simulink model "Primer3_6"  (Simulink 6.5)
settings: Solver=ode23t  SolverMode=SingleTasking  StartTime=0.0  StopTime=1  RelTol=1e-3  AbsTol=1e-2
undefined symbols (not defined in the file or in its folder): blocks, Continuous, powergui, ZData
libraries: powerlib x8, powerlib_extras x2

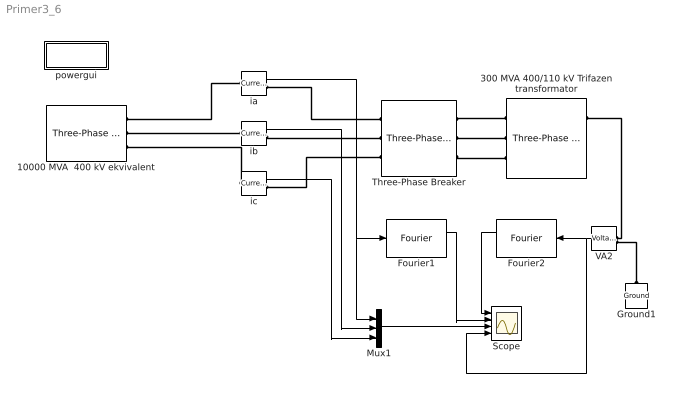
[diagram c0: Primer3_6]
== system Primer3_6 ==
  10000 MVA  400 kV ekvivalent : powerlib/Electrical Sources/Three-Phase Source  DialogController=PMDialogs.PMDefaultMaskDlg  SystemSampleTime=-1  Voltage=400e3  PhaseAngle=0  Frequency=50  InternalConnection=Yg  SpecifyImpedance=on  Resistance=5.55  Inductance=0.221  ShortCircuitLevel=10000e6  BaseVoltage=400e3  XRratio=10
  300 MVA 400/110 kV Trifazen transformator : powerlib/Elements/Three-Phase Transformer (Two Windings)  DialogController=PMDialogs.PMDefaultMaskDlg  SystemSampleTime=-1  UNITS=pu  NominalPower=[ 300e6 50 ]  Winding1Connection=Yg  Winding1=[ 400e3 0.0005 0.02 ]  Winding2Connection=Yg  Winding2=[ 115.5e3 0.0005 0.02]  SetSaturation=on  Rm=125  Lm=500  Saturation="[0 0; 0.0 1.2; 1.0  1.52]"  Hysteresis=off  DataFile='hysteresis'  SetInitialFlux=off  InitialFluxes=[-0.000666222505893204 0.000333111406701593 0.000333111099191611]  Measurements=None  TransfoNumber=0  MoreParameters=off  BreakLoop=off  DataType=off
  Fourier1 : powerlib_extras/Measurements/Fourier  DialogController=PMDialogs.PMDefaultMaskDlg  SystemSampleTime=-1  f1=50  n=3
  Fourier2 : powerlib_extras/Measurements/Fourier  Orientation=left  DialogController=PMDialogs.PMDefaultMaskDlg  SystemSampleTime=-1  f1=50  n=3
  Ground1 : powerlib/Elements/Ground  Orientation=down  DialogController=PMDialogs.PMDefaultMaskDlg  PhysicalDomain=powersysdomain  SubClassName=unknown  LeftPortType=p1  RightPortType=p1  LConnTagsString=a
  Mux1 : Mux  Inputs=3
  Scope : Scope  NumInputPorts=4
  Three-Phase Breaker : powerlib/Elements/Three-Phase Breaker  DialogController=PMDialogs.PMDefaultMaskDlg  SystemSampleTime=-1  InitialState=open  SwitchA=on  SwitchB=on  SwitchC=on  SwitchTimes=[0.05]  External=off  BreakerResistance=0.001  SnubberResistance=100e6  SnubberCapacitance=inf  Measurements=None
  VA2 : powerlib/Measurements/Voltage Measurement  Tag=PoWeRsYsTeMmEaSuReMeNt  Orientation=left  DialogController=PMDialogs.PMDefaultMaskDlg  SystemSampleTime=-1  PhasorSimulation=off  OutputType=Magnitude  PSBequivalent=0
  ia : powerlib/Measurements/Current Measurement  Tag=PoWeRsYsTeMmEaSuReMeNt  DialogController=PMDialogs.PMDefaultMaskDlg  SystemSampleTime=-1  PhasorSimulation=off  OutputType=Magnitude  PSBequivalent=0
  ib : powerlib/Measurements/Current Measurement  Tag=PoWeRsYsTeMmEaSuReMeNt  DialogController=PMDialogs.PMDefaultMaskDlg  SystemSampleTime=-1  PhasorSimulation=off  OutputType=Magnitude  PSBequivalent=0
  ic : powerlib/Measurements/Current Measurement  Tag=PoWeRsYsTeMmEaSuReMeNt  DialogController=PMDialogs.PMDefaultMaskDlg  SystemSampleTime=-1  PhasorSimulation=off  OutputType=Magnitude  PSBequivalent=0
  powergui : Subsystem  AncestorBlock=powerlib/powergui  InitFcn=powergui( 'InitFcn_Callback' , gcb , 0 , [ ] );  mask(PSB option menu block){SimulationMode=Continuous, SampleTime=0, echomessages=off, RestoreLinks=warning, x0status=blocks, Frange=[0:2:500], Ylog=off, Xlog=on, ShowGrid=off, save=off, variable=ZData, structure=, ZoomFFT=on, StartTime=0.0, cycles=1, DisplayStyle=1, fundamental=60, FreqAxis=off, MaxFrequency=1000, frequencyindice=50, frequencyindicesteady=1, RmsSteady=1, display=off, Ts=0, frequency=60, methode=off, HookPort=off, Interpol=off}
      mask prompts: SimulationMode "Simulation mode"; SampleTime "Sample time Ts (when simulation mode is Discrete) (s)"; echomessages "Echo  Messages"; RestoreLinks "Restore disabled links"; x0status "Initial electrical states status"; Frange "Impedance tool: Frequency Range"; Ylog "Impedance tool: Log impedance"; Xlog "Impedance tool: log Frequency"; ShowGrid "Impedance tool: grid"; save "Impedance tool: Save Data To Workspace"; variable "Impedance tool: Variable Name"; structure "Structure Name (PSBFFTSCOPE)"; ZoomFFT "ZoomFFT (PSBFFTSCOPE)"; StartTime "Start Time (PSBFFTSCOPE)"; cycles "Cycles (PSBFFTSCOPE)"; DisplayStyle "Display style (PSBFFTSCOPE)"; fundamental "Fundamental (PSBFFTSCOPE)"; FreqAxis "Frequency Axis (PSBFFTSCOPE)"; MaxFrequency "Max Frequency (PSBFFTSCOPE)"; frequencyindice "Load flow frequency (Hz)"; frequencyindicesteady "Frequency indice (STEADYSTATE)"; RmsSteady "RMS display (STEADYSTATE)"; display "Display Results"; Ts "OBSOLETE 1"; frequency "Phasor frequency (Hz)"; methode "Phasor simulation"; HookPort "Hook port"; Interpol "Interpolate"
      mask init:
      | powerlibroot = which('powersysdomain');
      | PSBroot = powerlibroot(1:end-16);
      | %
      | switch SimulationMode
      | 	case 1
      | 		message=sprintf('Continuous');
      | 	case 2
      |         SampleTimeeval=evalin('base',SampleTime,'NaN');
      |         if isnan(SampleTimeeval)
      |             message=sprintf('Warning !!,\nUndefined sample time');
      |         else
      |             message=sprintf('Discrete,\nTs = %.4g s.',SampleTimeeval);
      |         end
      | 	case 3
      | 		message=sprintf('Phasors');
      | end
      | if strcmp(bdroot,'powerlib')
      |   message='powergui';
      | end
      | power_initmask();
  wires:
  ia/1 -> Mux1/1, Fourier1/1
  ib/1 -> Mux1/2
  ic/1 -> Mux1/3
  Fourier1/1 -> Scope/2
  VA2/1 -> Fourier2/1, Scope/4
  Fourier2/1 -> Scope/1
  Mux1/1 -> Scope/3
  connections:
  ic/LConn1 -- 10000 MVA  400 kV ekvivalent/RConn3
  ib/LConn1 -- 10000 MVA  400 kV ekvivalent/RConn2
  300 MVA 400/110 kV Trifazen transformator/RConn1 -- VA2/LConn1
  10000 MVA  400 kV ekvivalent/RConn1 -- ia/LConn1
  Three-Phase Breaker/RConn1 -- 300 MVA 400/110 kV Trifazen transformator/LConn1
  Three-Phase Breaker/RConn2 -- 300 MVA 400/110 kV Trifazen transformator/LConn2
  Three-Phase Breaker/RConn3 -- 300 MVA 400/110 kV Trifazen transformator/LConn3
  ia/RConn1 -- Three-Phase Breaker/LConn1
  ib/RConn1 -- Three-Phase Breaker/LConn2
  ic/RConn1 -- Three-Phase Breaker/LConn3
  Ground1/LConn1 -- VA2/LConn2

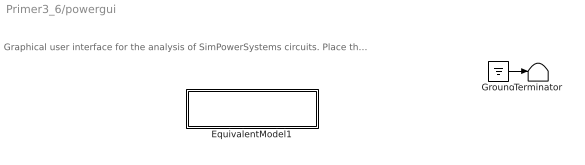
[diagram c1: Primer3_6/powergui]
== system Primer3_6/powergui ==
  note: Graphical user interface for the analysis of SimPowerSystems circuits. Place the Powergui block in the top-level of your model and double-click on it to open the GUI.
  EquivalentModel1 : Subsystem
  Ground : Ground
  Terminator : Terminator
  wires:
  Ground/1 -> Terminator/1

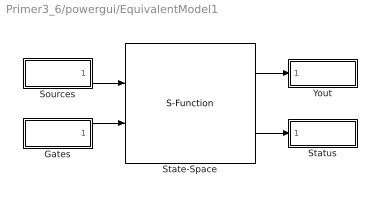
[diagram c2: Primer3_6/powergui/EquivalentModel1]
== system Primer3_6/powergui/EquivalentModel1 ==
  Gates : Subsystem
  Sources : Subsystem
  State-Space : S-Function  FunctionName=sfun_spssw_contc  Parameters=A, B, C, D, x0, SwitchResistance ,SwitchType, SwitchGateInitialValue, OutputsToResetToZero
  Status : Subsystem
  Yout : Subsystem
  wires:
  Gates/1(gates) -> State-Space/2
  Sources/1(u) -> State-Space/1
  State-Space/2 -> Status/1(status)
  State-Space/1 -> Yout/1(v,i)

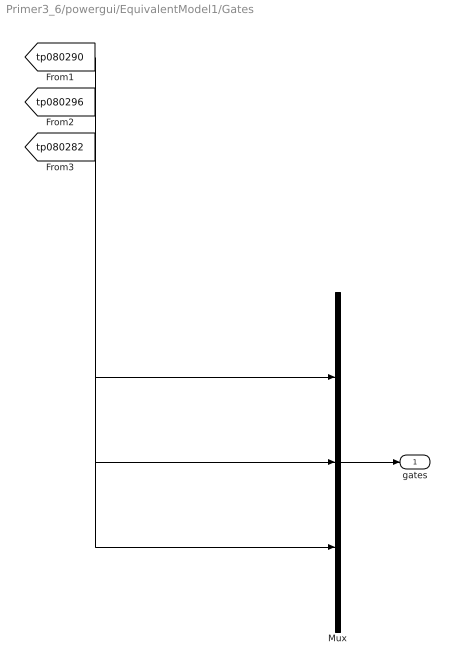
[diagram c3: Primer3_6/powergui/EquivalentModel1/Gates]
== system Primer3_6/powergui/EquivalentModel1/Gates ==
  Mux : Mux  Inputs=[1 1 1]
  gates : Outport
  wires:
  Mux/1 -> gates/1
  [tp080290] -> Mux/1
  [tp080296] -> Mux/2
  [tp080282] -> Mux/3

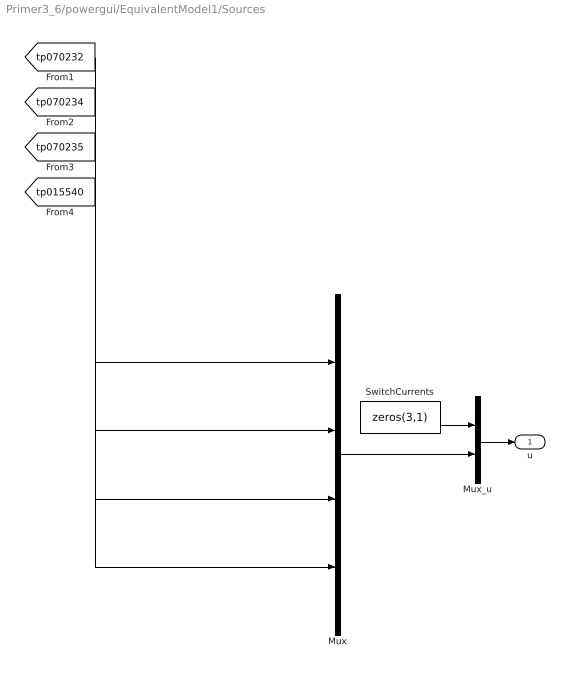
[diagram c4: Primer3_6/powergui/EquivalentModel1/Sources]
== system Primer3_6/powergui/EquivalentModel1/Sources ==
  Mux : Mux  Inputs=[1 1 1 3]
  Mux_u : Mux  Inputs=[3 6]
  SwitchCurrents : Constant  Value=zeros(3,1)  OutDataType=sfix(16)  ConRadixGroup=Use specified scaling  OutScaling=2^0  SampleTime=inf  FramePeriod=inf
  u : Outport
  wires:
  Mux/1 -> Mux_u/2
  SwitchCurrents/1 -> Mux_u/1
  Mux_u/1 -> u/1
  [tp070232] -> Mux/1
  [tp070234] -> Mux/2
  [tp070235] -> Mux/3
  [tp015540] -> Mux/4

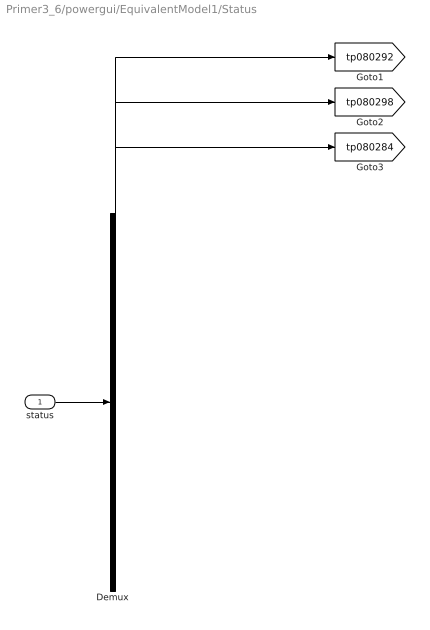
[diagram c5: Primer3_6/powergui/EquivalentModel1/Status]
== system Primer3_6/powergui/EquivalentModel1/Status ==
  status : Inport
  Demux : Demux  Outputs=[1 1 1]
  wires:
  status/1 -> Demux/1
  Demux/1 -> [tp080292]
  Demux/2 -> [tp080298]
  Demux/3 -> [tp080284]

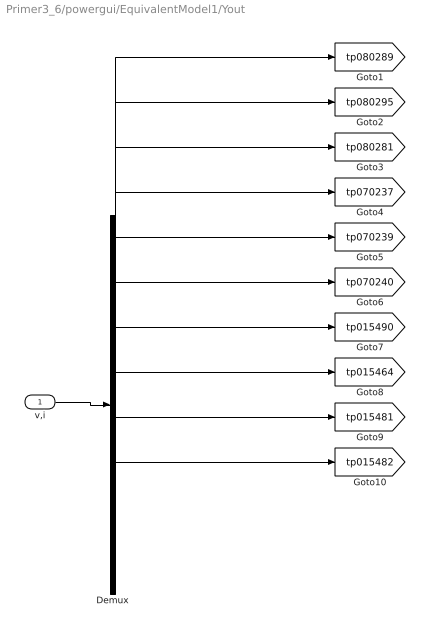
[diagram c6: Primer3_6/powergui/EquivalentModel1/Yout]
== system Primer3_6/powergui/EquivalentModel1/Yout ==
  v,i : Inport
  Demux : Demux  Outputs=[1 1 1 1 1 1 1 1 1 1]
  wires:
  v,i/1 -> Demux/1
  Demux/1 -> [tp080289]
  Demux/2 -> [tp080295]
  Demux/3 -> [tp080281]
  Demux/4 -> [tp070237]
  Demux/5 -> [tp070239]
  Demux/6 -> [tp070240]
  Demux/7 -> [tp015490]
  Demux/8 -> [tp015464]
  Demux/9 -> [tp015481]
  Demux/10 -> [tp015482]
